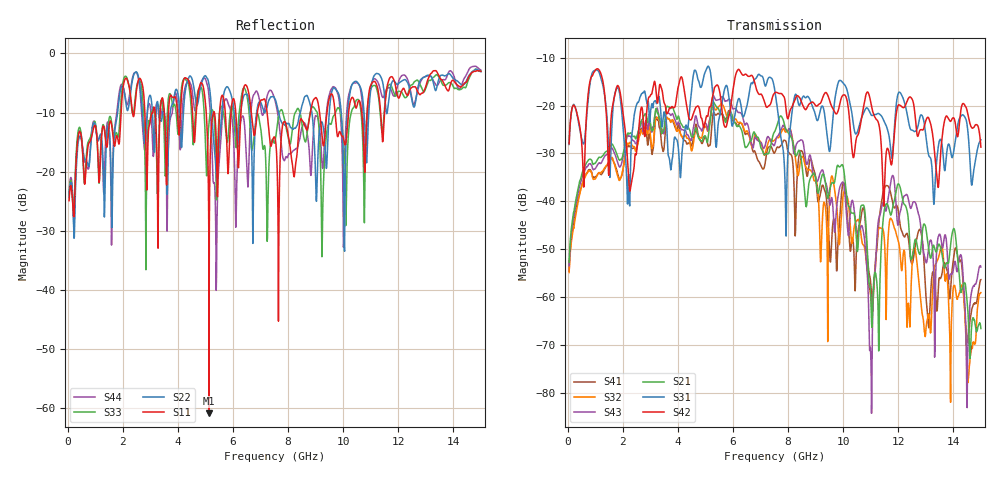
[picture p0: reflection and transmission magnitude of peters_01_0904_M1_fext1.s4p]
# MHZ S RI R 50.00
! FREQ  S11  S12  S13  S14
!  S21  S22  S23  S24
!  S31  S32  S33  S34
!  S41  S42  S43  S44
!  REAL  IMAG  REAL  IMAG  REAL  IMAG  REAL  IMAG
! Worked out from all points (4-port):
!   1496 points, 50 MHz to 15 GHz, reference 50 ohm
!   strongest paths, dB at 50 MHz, 3.79 GHz, 7.53 GHz, 11.27 GHz, 15 GHz:
!     S42: -28.0, -20.2, -17.3, -23.4, -28.7
!     S31: -28.1, -31.3, -17.3, -21.7, -27.2
!     S21: -52.7, -20.3, -25.3, -63.4, -66.6
!     S43: -53.5, -21.7, -27.9, -44.4, -53.7
!     S32: -54.9, -23.0, -27.1, -46.2, -59.1
!     S41: -54.6, -23.1, -29.7, -46.1, -56.4
!   lowest |S11| = -60.9 dB at 5.13 GHz (marker M1), VSWR 1.00, Z = 50.1 - j0.0139 ohm
!   |S11| at or under -10 dB: start of sweep to 1.937 GHz; 7.237 GHz to 8.809 GHz (1.572 GHz wide, 19.6 % of centre); 9.707 GHz to 10.2 GHz (489.4 MHz wide, 4.92 % of centre)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
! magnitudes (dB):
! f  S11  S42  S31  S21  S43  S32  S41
! 50 MHz  -24.9  -28.0  -28.1  -52.7  -53.5  -54.9  -54.6
! 5.13 GHz  -60.9  -20.6  -12.0  -25.2  -23.7  -23.6  -28.4
! 7.91 GHz  -11.8  -19.9  -42.1  -24.8  -25.0  -25.6  -27.4
! 9.98 GHz  -14.0  -17.9  -15.2  -32.4  -36.0  -39.7  -36.5
! 11 GHz  -5.4  -19.3  -21.8  -59.6  -72.0  -59.7  -57.1
! 11.78 GHz  -4.0  -31.6  -31.0  -41.8  -34.7  -44.1  -39.8
! 15 GHz  -3.0  -28.7  -27.2  -66.6  -53.7  -59.1  -56.4
